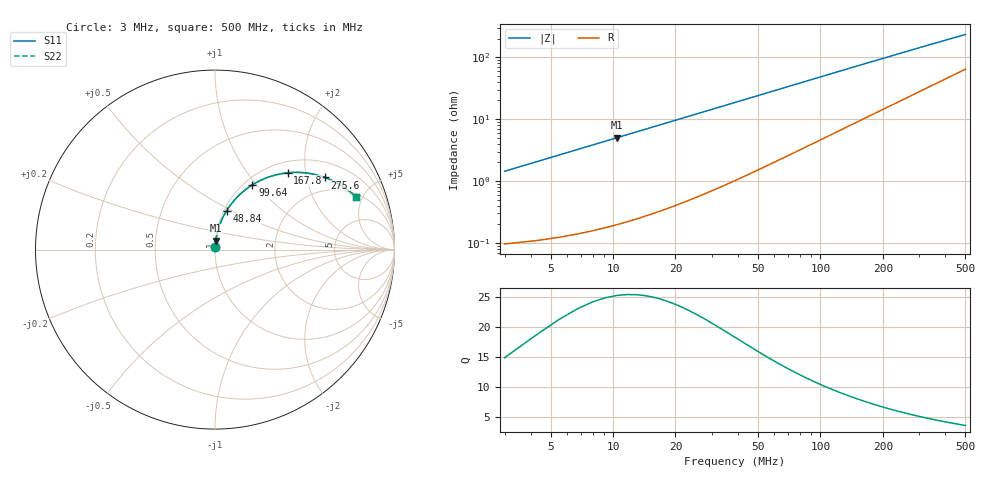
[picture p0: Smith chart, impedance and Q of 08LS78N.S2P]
! Coilcraft 0805LS-78N Chip Inductor
! 18 September 2002
# MHZ S MA R 50
!Freq  MagS11  AngS11  MagS21  AngS21  MagS12  AngS12  MagS22  AngS22
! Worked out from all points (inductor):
!   403 points, 3 MHz to 500 MHz, reference 50 ohm
!   read as one part in series: L = 76.2 nH near 5.478 MHz
!   highest Q = 25 at 10.43 MHz (marker M1), where L = 76.2 nH
!   S11 on the Smith chart (normalised r, x): 3 MHz: 1.00, +0.03; 48.84 MHz: 1.03, +0.47; 99.64 MHz: 1.09, +0.95; 167.8 MHz: 1.22, +1.59; 275.6 MHz: 1.48, +2.57; 500 MHz: 2.27, +4.47
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3  0.01438 85.3  0.9989 -0.8  0.9989 -0.8  0.01438 85.3
4.239  0.0203 85.8  0.9987 -1.2  0.9987 -1.2  0.0203 85.8
7.956  0.03803 85.5  0.9977 -2.2  0.9977 -2.2  0.03803 85.5
10.434  0.04984 84.9  0.9968 -2.9  0.9968 -2.9  0.04984 84.9
12.912  0.06161 84.2  0.9957 -3.5  0.9957 -3.5  0.06161 84.2
16.629  0.07922 83.1  0.9937 -4.5  0.9937 -4.5  0.07922 83.1
20.346  0.09673 82.0  0.9912 -5.5  0.9912 -5.5  0.09673 82.0
25.302  0.1199 80.5  0.9874 -6.9  0.9874 -6.9  0.1199 80.5
35.214  0.1654 77.5  0.9776 -9.5  0.9776 -9.5  0.1654 77.5
48.843  0.2255 73.4  0.9604 -13.0  0.9604 -13.0  0.2255 73.4
66.189  0.297 68.5  0.9331 -17.2  0.9331 -17.2  0.297 68.5
86.013  0.3709 63.3  0.8969 -21.7  0.8969 -21.7  0.3709 63.3
99.642  0.4166 60.0  0.87 -24.5  0.87 -24.5  0.4166 60.0
130.617  0.5057 53.3  0.807 -30.2  0.807 -30.2  0.5057 53.3
167.787  0.5889 46.6  0.7332 -35.7  0.7332 -35.7  0.5889 46.6
169.026  0.5913 46.4  0.7308 -35.9  0.7308 -35.9  0.5913 46.4
209.913  0.6586 40.5  0.6573 -40.6  0.6573 -40.6  0.6586 40.5
252.039  0.7095 35.6  0.5917 -44.3  0.5917 -44.3  0.7095 35.6
275.58  0.7319 33.3  0.5593 -46.0  0.5593 -46.0  0.7319 33.3
335.052  0.7749 28.6  0.4896 -49.2  0.4896 -49.2  0.7749 28.6
418.065  0.814 23.8  0.4155 -52.1  0.4155 -52.1  0.814 23.8
500  0.8388 20.3  0.361 -53.8  0.361 -53.8  0.8388 20.3
